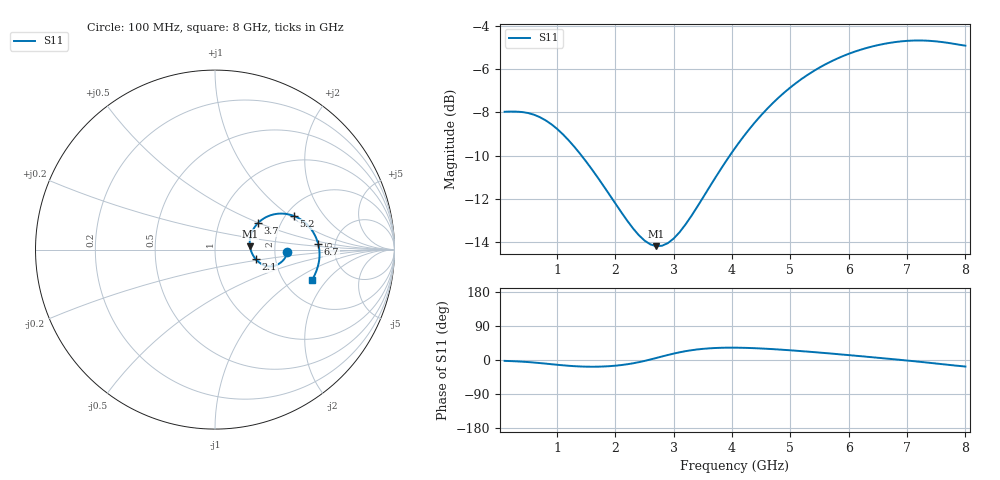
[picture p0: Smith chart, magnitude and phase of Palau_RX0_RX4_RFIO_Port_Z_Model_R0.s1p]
! Created Fri Jul 17 10:29:10 2020
! Palau RX0/RX4 RFIO Port Impedance Model.
! Revision		: R0.
! Impedance Mode 	: Balanced Differential-Mode.
! Impedance Format 	: Series Equivalent Differential Impedance (SEDZ).
# hz S ma R 50
! 1 Port Network Data from SP1.SP block
! freq  magS11  angS11
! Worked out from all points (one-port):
!   80 points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, 100 MHz to 8 GHz, reference 50 ohm
!   lowest |S11| = -14.2 dB at 2.7 GHz (marker M1), VSWR 1.49, Z = 74.1 + j2.79 ohm
!   |S11| at or under -10 dB: 1.42 GHz to 3.96 GHz (2.541 GHz wide, 94.5 % of centre)
!   S11 on the Smith chart (normalised r, x): 100 MHz: 2.33, -0.09; 2.1 GHz: 1.58, -0.18; 3.7 GHz: 1.53, +0.49; 5.2 GHz: 2.20, +1.07; 6.7 GHz: 3.68, +0.33; 8 GHz: 2.85, -1.42
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1e8  0.3994 -2.3
4e8  0.3988 -4.4
6e8  0.3934 -6.6
8e8  0.3818 -9.5
1.1e9  0.3542 -14.0
1.3e9  0.331 -16.4
1.6e9  0.2936 -17.8
1.8e9  0.2687 -17.1
2.1e9  0.2342 -13.4
2.4e9  0.2073 -5.8
2.6e9  0.1973 1.3
2.7e9  0.1954 5.3
2.9e9  0.1987 13.3
3.1e9  0.2105 20.3
3.4e9  0.2406 27.8
3.7e9  0.2795 31.6
4.1e9  0.3364 32.4
4.4e9  0.3787 31.1
4.6e9  0.4056 29.6
5.1e9  0.4657 24.4
5.2e9  0.4763 23.3
5.6e9  0.5139 18.3
6.1e9  0.5497 11.5
6.4e9  0.565 7.3
6.7e9  0.576 3.0
7.1e9  0.5832 -2.9
7.5e9  0.5806 -9.3
8e9  0.5676 -17.3
